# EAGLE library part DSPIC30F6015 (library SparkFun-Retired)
Microchip 16-bit DSP SparkFun Products None
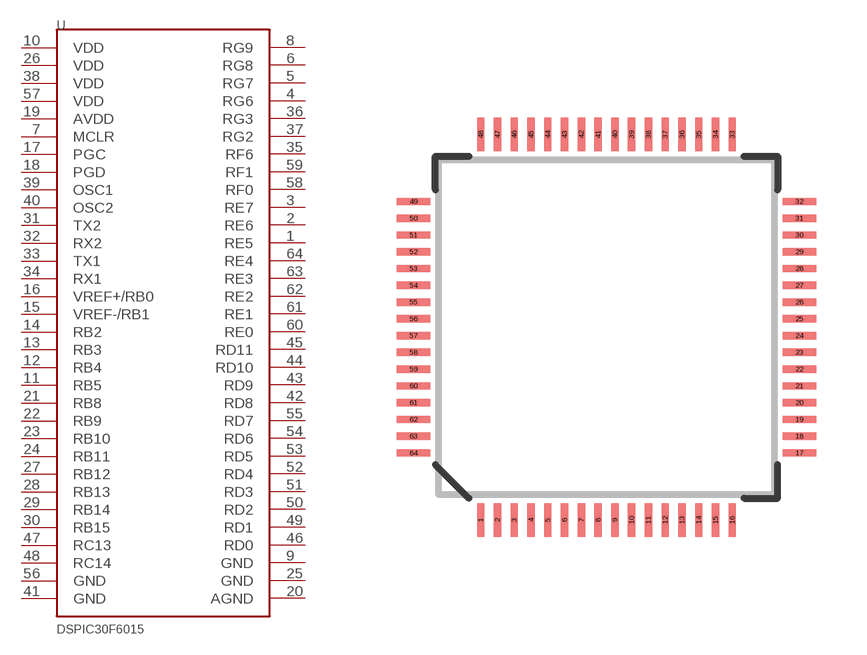
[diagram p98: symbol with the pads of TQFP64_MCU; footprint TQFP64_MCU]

Designator prefix U

## DSPIC30F6015SMD  [TQFP64_MCU]
1  RE5
2  RE6
3  RE7
4  RG6
5  RG7
6  RG8
7  MCLR
8  RG9
9  GND
10  VDD
11  RB5
12  RB4
13  RB3
14  RB2
15  VREF-/RB1
16  VREF+/RB0
17  PGC
18  PGD
19  AVDD
20  AGND
21  RB8
22  RB9
23  RB10
24  RB11
25  GND
26  VDD
27  RB12
28  RB13
29  RB14
30  RB15
31  TX2
32  RX2
33  TX1
34  RX1
35  RF6
36  RG3
37  RG2
38  VDD
39  OSC1
40  OSC2
41  GND
42  RD8
43  RD9
44  RD10
45  RD11
46  RD0
47  RC13
48  RC14
49  RD1
50  RD2
51  RD3
52  RD4
53  RD5
54  RD6
55  RD7
56  GND
57  VDD
58  RF0
59  RF1
60  RE0
61  RE1
62  RE2
63  RE3
64  RE4

## Footprint TQFP64_MCU (pad centres in mm)
64-Lead TQFP Plastic Thin Quad Flatpack - 10x10x1mm Body, 2mmFP
smd 0.22 x 1: 1 -3.75,-5.75; 2 -3.25,-5.75; 3 -2.75,-5.75; 4 -2.25,-5.75; 5 -1.75,-5.75; 6 -1.25,-5.75; 7 -0.75,-5.75; 8 -0.25,-5.75; 9 0.25,-5.75; 10 0.75,-5.75; 11 1.25,-5.75; 12 1.75,-5.75; 13 2.25,-5.75; 14 2.75,-5.75; 15 3.25,-5.75; 16 3.75,-5.75; 33 3.75,5.75; 34 3.25,5.75; 35 2.75,5.75; 36 2.25,5.75; 37 1.75,5.75; 38 1.25,5.75; 39 0.75,5.75; 40 0.25,5.75; 41 -0.25,5.75; 42 -0.75,5.75; 43 -1.25,5.75; 44 -1.75,5.75; 45 -2.25,5.75; 46 -2.75,5.75; 47 -3.25,5.75; 48 -3.75,5.75
smd 1 x 0.22: 17 5.75,-3.75; 18 5.75,-3.25; 19 5.75,-2.75; 20 5.75,-2.25; 21 5.75,-1.75; 22 5.75,-1.25; 23 5.75,-0.75; 24 5.75,-0.25; 25 5.75,0.25; 26 5.75,0.75; 27 5.75,1.25; 28 5.75,1.75; 29 5.75,2.25; 30 5.75,2.75; 31 5.75,3.25; 32 5.75,3.75; 49 -5.75,3.75; 50 -5.75,3.25; 51 -5.75,2.75; 52 -5.75,2.25; 53 -5.75,1.75; 54 -5.75,1.25; 55 -5.75,0.75; 56 -5.75,0.25; 57 -5.75,-0.25; 58 -5.75,-0.75; 59 -5.75,-1.25; 60 -5.75,-1.75; 61 -5.75,-2.25; 62 -5.75,-2.75; 63 -5.75,-3.25; 64 -5.75,-3.75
